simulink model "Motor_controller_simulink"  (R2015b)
settings: Solver=ode5  StartTime=0.0  StopTime=10.0  FixedStep=0.001  RelTol=1e-3

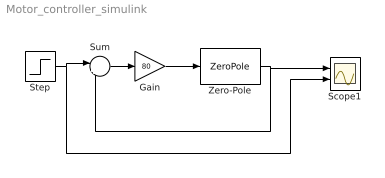
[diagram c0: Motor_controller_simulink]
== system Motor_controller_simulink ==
  Gain : Gain  Gain=80
  Scope1 : Scope  NumInputPorts=2
  Step : Step  Time=0  SampleTime=0
  Sum : Sum  Inputs=|+-
  Zero-Pole : ZeroPole  Zeros=[]  Poles=[0 -8]
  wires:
  Sum/1 -> Gain/1
  Gain/1 -> Zero-Pole/1
  Zero-Pole/1 -> Scope1/1, Sum/2
  Step/1 -> Scope1/2, Sum/1
